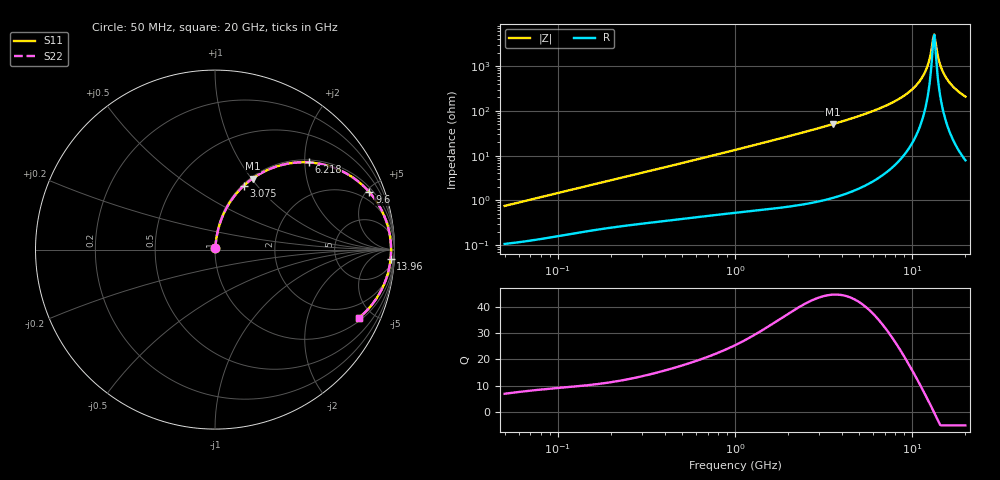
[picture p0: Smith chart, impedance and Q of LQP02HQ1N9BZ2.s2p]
!Murata Part Number: LQP02HQ1N9BZ2
!These Parameters are Measured in Series Mode Connection
!  o--[Z]--o
!Port1  Port2
!  o-------o
!Freq. Start=50[MHz] Stop=20[GHz], 401[Steps]
# Hz S RI R 50
!Freq.(Hz) S11(Real) S11(Imag) S21(Real) S21(Imag) S12(Real) S12(Imag) S22(Real) S22(Imag)
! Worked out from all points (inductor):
!   401 points, 50 MHz to 20 GHz, reference 50 ohm
!   read as one part in series: L = 2.36 nH near 51.52 MHz
!   highest Q = 44.5 at 3.572 GHz (marker M1), where L = 2.26 nH
!   self-resonance near 13.15 GHz
!   S11 on the Smith chart (normalised r, x): 50 MHz: 1.00, +0.01; 3.075 GHz: 1.02, +0.85; 6.218 GHz: 1.06, +2.09; 9.6 GHz: 1.29, +5.25; 13.96 GHz: 12, -32; 20 GHz: 1.16, -4.16
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5e7  0.00112 0.00743  0.9989 -0.00743  0.9989 -0.00743  0.00112 0.00743
1.364002e8  0.00233 0.0194  0.9977 -0.0194  0.9977 -0.0194  0.00233 0.0194
3.721004e8  0.00589 0.0504  0.9941 -0.0504  0.9941 -0.0504  0.00589 0.0504
1e9  0.0226 0.1301  0.9774 -0.1301  0.9774 -0.1301  0.0226 0.1301
2.728004e9  0.129 0.3236  0.871 -0.3236  0.871 -0.3236  0.129 0.3236
3.075291e9  0.1601 0.3555  0.8399 -0.3555  0.8399 -0.3555  0.1601 0.3555
3.572216e9  0.2093 0.3957  0.7907 -0.3957  0.7907 -0.3957  0.2093 0.3957
6.217679e9  0.5214 0.486  0.4786 -0.486  0.4786 -0.486  0.5214 0.486
7.442007e9  0.664 0.4558  0.336 -0.4558  0.336 -0.4558  0.664 0.4558
9.600142e9  0.8602 0.3201  0.1398 -0.3201  0.1398 -0.3201  0.8602 0.3201
1.066139e10  0.9223 0.2309  0.0777 -0.2309  0.0777 -0.2309  0.9223 0.2309
1.166392e10  0.9595 0.142  0.0405 -0.142  0.0405 -0.142  0.9595 0.142
1.238412e10  0.9745 0.0783  0.0255 -0.0783  0.0255 -0.0783  0.9745 0.0783
1.295331e10  0.9801 0.0293  0.0199 -0.0293  0.0199 -0.0293  0.9801 0.0293
1.314879e10  0.9809 0.0128  0.0191 -0.0128  0.0191 -0.0128  0.9809 0.0128
1.334722e10  0.9811 -0.00374  0.0189 0.00374  0.0189 0.00374  0.9811 -0.00374
1.354865e10  0.9808 -0.0202  0.0192 0.0202  0.0192 0.0202  0.9808 -0.0202
1.396067e10  0.9784 -0.0531  0.0216 0.0531  0.0216 0.0531  0.9784 -0.0531
1.460232e10  0.9708 -0.1019  0.0292 0.1019  0.0292 0.1019  0.9708 -0.1019
1.573793e10  0.9475 -0.1799  0.0525 0.1799  0.0525 0.1799  0.9475 -0.1799
1.747767e10  0.8955 -0.2783  0.1045 0.2783  0.1045 0.2783  0.8955 -0.2783
2e10  0.8036 -0.3788  0.1964 0.3788  0.1964 0.3788  0.8036 -0.3788
